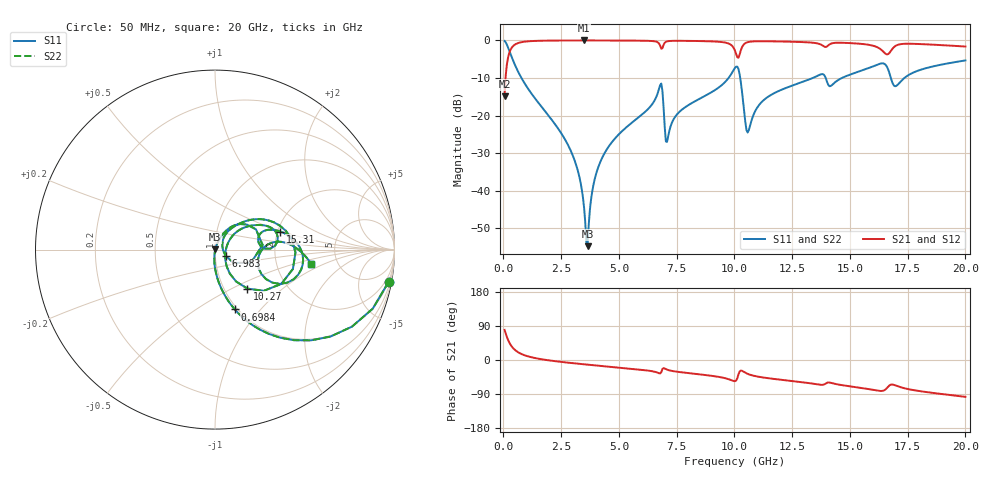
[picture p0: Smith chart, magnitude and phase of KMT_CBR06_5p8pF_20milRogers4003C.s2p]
! Data measured by Modelithics Inc. support@modelithics.com 813-866-6335
! KEMET CBR0603 5.8pF, Pad Width= 0.851mm, Pad Length= 0.64mm, Pad Gap= 0.62mm, 20mil Rogers 4003C substrate Data, January 2022
# hz S ma R 50
! 2 Port Network Data from SP1.SP block
! freq  magS11  angS11  magS21  angS21  magS12  angS12  magS22  angS22
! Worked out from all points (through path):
!   401 points, 50 MHz to 20 GHz, reference 50 ohm
!   highest |S21| = -0.01 dB at 3.491 GHz (marker M1); lowest = -14.9 dB at 50 MHz (marker M2)
!   group delay of S21, straight-line fit = 15 ps
!   lowest |S11| = -54.7 dB at 3.641 GHz (marker M3), VSWR 1.00, Z = 50.2 + j0.0574 ohm
!   |S11| at or under -10 dB: 779.9 MHz to 9.745 GHz (8.965 GHz wide, 170 % of centre); 10.25 GHz to 13.39 GHz (3.141 GHz wide, 26.6 % of centre); 13.95 GHz to 14.65 GHz (701.2 MHz wide, 4.9 % of centre)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
!   |S22| runs from -54.7 to -0.1 dB; largest |S21 - S12| = 0
!   S11 on the Smith chart (normalised r, x): 50 MHz: 1, -11; 698.4 MHz: 0.97, -0.74; 6.983 GHz: 1.12, -0.08; 10.27 GHz: 1.28, -0.61; 15.31 GHz: 2.07, +0.48; 20 GHz: 3.19, -0.71
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5e7  0.9835 -10.6  0.1808 79.4  0.1808 79.4  0.9835 -10.6
2.99375e8  0.6698 -48.9  0.7419 41.0  0.7419 41.0  0.6698 -48.9
6.98375e8  0.3516 -71.6  0.9354 18.2  0.9354 18.2  0.3516 -71.6
2.74325e9  0.04359 -94.9  0.9976 -6.7  0.9976 -6.7  0.04359 -94.9
3.391625e9  0.01043 -92.4  0.9983 -10.8  0.9983 -10.8  0.01043 -92.4
3.491375e9  0.005949 -86.3  0.9983 -11.4  0.9983 -11.4  0.005949 -86.3
3.641e9  0.001834 18.2  0.9983 -12.3  0.9983 -12.3  0.001834 18.2
3.94025e9  0.01383 69.1  0.9981 -14.0  0.9981 -14.0  0.01383 69.1
4.33925e9  0.03011 70.4  0.9976 -16.2  0.9976 -16.2  0.03011 70.4
6.73325e9  0.2252 38.4  0.9115 -34.9  0.9115 -34.9  0.2252 38.4
6.982625e9  0.07034 -31.1  0.9301 -22.7  0.9301 -22.7  0.07034 -31.1
7.13225e9  0.05337 39.9  0.9772 -26.6  0.9772 -26.6  0.05337 39.9
7.581125e9  0.1093 55.3  0.9876 -31.5  0.9876 -31.5  0.1093 55.3
1.0025e10  0.4319 7.5  0.7288 -55.9  0.7288 -55.9  0.4319 7.5
1.027438e10  0.2827 -50.3  0.7326 -27.8  0.7326 -27.8  0.2827 -50.3
1.057362e10  0.05959 -6.9  0.9475 -36.6  0.9475 -36.6  0.05959 -6.9
1.137162e10  0.1706 39.0  0.974 -47.3  0.974 -47.3  0.1706 39.0
1.336662e10  0.3138 25.0  0.9334 -62.1  0.9334 -62.1  0.3138 25.0
1.531175e10  0.3782 15.3  0.9088 -72.2  0.9088 -72.2  0.3782 15.3
1.670825e10  0.369 -29.9  0.6805 -67.2  0.6805 -67.2  0.369 -29.9
1.750625e10  0.3415 7.2  0.9034 -76.6  0.9034 -76.6  0.3415 7.2
2e10  0.5417 -8.4  0.8285 -97.2  0.8285 -97.2  0.5417 -8.4
